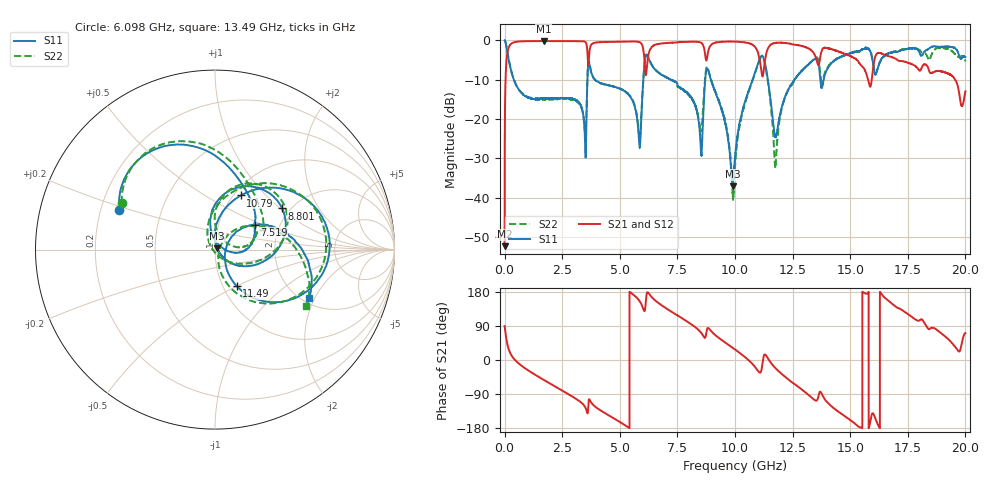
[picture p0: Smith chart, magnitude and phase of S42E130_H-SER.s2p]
! Created Wed Nov 25 21:58:15 2020
# khz S ma R 50
! 2 Port Network Data from SP1.SP block
! freq  magS11  angS11  magS21  angS21  magS12  angS12  magS22  angS22
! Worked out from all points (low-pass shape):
!   20001 points, 300 kHz to 20 GHz, reference 50 ohm
!   highest |S21| = -0.15 dB at 1.697 GHz (marker M1); lowest = -52.4 dB at 300 kHz (marker M2)
!   |S21| within 3 dB of the highest: 121.1 MHz to 3.596 GHz (3.475 GHz wide, 187 % of centre); 6.263 GHz to 8.694 GHz (2.431 GHz wide, 32.5 % of centre)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
!   lowest |S11| = -37.1 dB at 9.902 GHz (marker M3), VSWR 1.03, Z = 51.3 + j0.641 ohm
!   |S11| at or under -10 dB: 402.7 MHz to 3.594 GHz (3.192 GHz wide, 160 % of centre); 3.932 GHz to 6.02 GHz (2.089 GHz wide, 42 % of centre); 8.956 GHz to 10.76 GHz (1.806 GHz wide, 18.3 % of centre)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
!   |S22| runs from -40.6 to 0.0 dB; largest |S21 - S12| = 0.018
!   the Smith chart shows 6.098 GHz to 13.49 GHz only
!   S11 on the Smith chart (normalised r, x): 6.098 GHz: 0.28, +0.18; 7.519 GHz: 1.49, +0.44; 8.801 GHz: 1.82, +1.03; 10.79 GHz: 1.08, +0.73; 11.49 GHz: 1.16, -0.50; 13.49 GHz: 2.19, -1.80
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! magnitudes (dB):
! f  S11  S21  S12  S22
! 300 kHz  0.0  -52.4  -52.3  0.0
! 103.3 MHz  -2.3  -3.9  -3.9  -2.3
! 192.3 MHz  -5.3  -1.6  -1.6  -5.2
! 1.697 GHz  -14.8  -0.2  -0.2  -15.0
! 3.334 GHz  -16.9  -0.2  -0.2  -17.1
! 3.482 GHz  -24.2  -0.3  -0.3  -23.1
! 3.701 GHz  -6.7  -2.0  -2.0  -6.6
! 5.84 GHz  -26.0  -0.4  -0.4  -24.3
! 6.098 GHz  -4.8  -7.2  -7.2  -4.7
! 6.667 GHz  -8.2  -0.9  -0.9  -8.1
! 7.519 GHz  -11.7  -0.4  -0.5  -11.7
! 8.515 GHz  -27.1  -0.5  -0.6  -22.9
! 8.801 GHz  -7.2  -3.9  -3.9  -6.8
! 9.902 GHz  -37.1  -0.3  -0.3  -39.7
! 10 GHz  -29.8  -0.3  -0.3  -32.1
! 10.79 GHz  -9.5  -1.2  -1.2  -9.8
! 11.49 GHz  -12.5  -1.4  -1.5  -13.2
! 11.77 GHz  -24.6  -0.6  -0.6  -31.7
! 13.33 GHz  -5.3  -2.6  -2.6  -5.2
! 13.49 GHz  -4.6  -4.1  -4.1  -4.5
! 16.67 GHz  -3.3  -4.0  -4.2  -3.4
! 20 GHz  -4.2  -12.9  -12.8  -5.3
